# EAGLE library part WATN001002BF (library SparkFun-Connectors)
connector for 10x2 16-segment E-paper Display (LCD-10150) ***Unproven!!!***
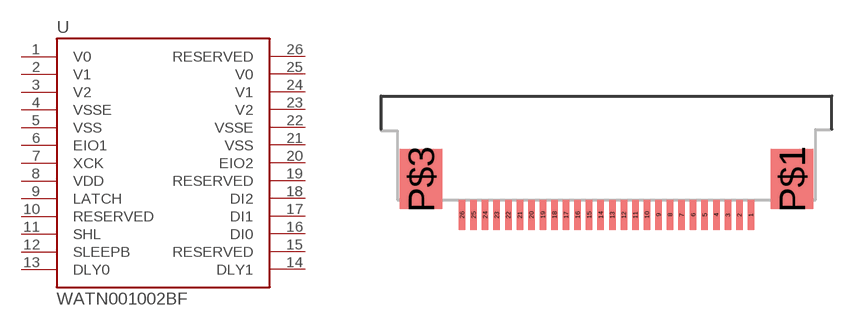
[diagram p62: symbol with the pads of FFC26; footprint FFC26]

Designator prefix U

## WATN001002BF  [FFC26]
1  V0
2  V1
3  V2
4  VSSE
5  VSS
6  EIO1
7  XCK
8  VDD
9  LATCH
10  RESERVED
11  SHL
12  SLEEPB
13  DLY0
14  DLY1
15  RESERVED
16  DI0
17  DI1
18  DI2
19  RESERVED
20  EIO2
21  VSS
22  VSSE
23  V2
24  V1
25  V0
26  RESERVED

## Footprint FFC26 (pad centres in mm)
26-pin FFC connector See 4UCONN part #08630
smd 0.28 x 1.3: 1 6.25,0; 2 5.75,0; 3 5.25,0; 4 4.75,0; 5 4.25,0; 6 3.75,0; 7 3.25,0; 8 2.75,0; 9 2.25,0; 10 1.75,0; 11 1.25,0; 12 0.75,0; 13 0.25,0; 14 -0.25,0; 15 -0.75,0; 16 -1.25,0; 17 -1.75,0; 18 -2.25,0; 19 -2.75,0; 20 -3.25,0; 21 -3.75,0; 22 -4.25,0; 23 -4.75,0; 24 -5.25,0; 25 -5.75,0; 26 -6.25,0
smd 1.85 x 2.6: P$1 8.025,1.55; P$3 -8.025,1.55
